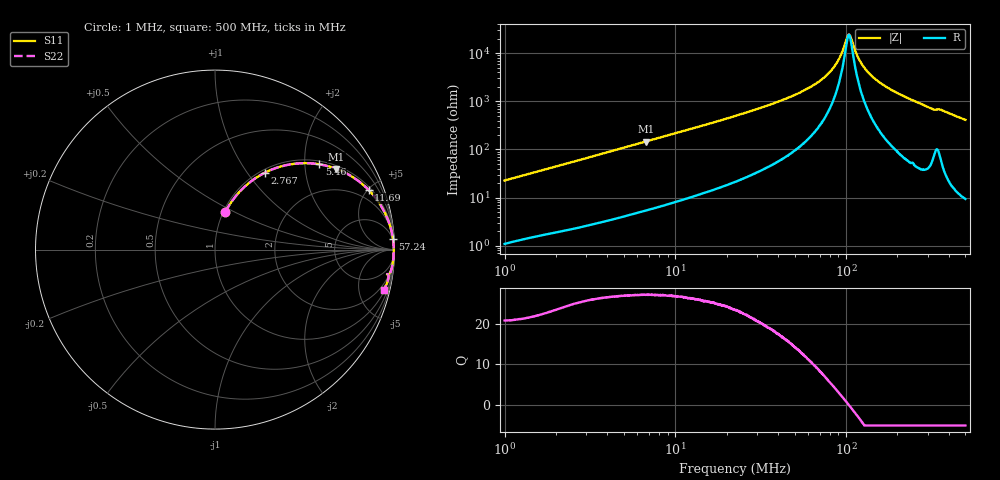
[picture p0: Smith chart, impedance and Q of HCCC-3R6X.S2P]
!s-Parameter Generated by FASTRON Sdn. Bhd.
!FASTRON P/N : HCCC-3R6X
!Keysight Technologies,E4991B,MY54100416,A.01.15
!Date: Thu Apr 02 14:45:55 2026
!Version  : Rev00 Thu Apr 02 14:45:55 2026
!Data & Calibration Information:
!PortZ  Port1:50+j0  Port2:50+j0
!When reading, reference impedance value at option line is always used.
!Remarks : This data is being provided solely for informational purposes.
!Freq	S11	S21	S12	S22
# Hz S dB R 50
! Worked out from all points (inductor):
!   1601 points, 1 MHz to 500 MHz, reference 50 ohm
!   read as one part in series: L = 3.57 uH near 1.032 MHz
!   highest Q = 27.1 at 6.76 MHz (marker M1), where L = 3.45 uH
!   self-resonance near 103.7 MHz
!   S11 on the Smith chart (normalised r, x): 1 MHz: 1.02, +0.45; 2.767 MHz: 1.05, +1.22; 5.46 MHz: 1.09, +2.37; 11.69 MHz: 1.19, +5.05; 57.24 MHz: 4, +34; 500 MHz: 1.19, -8.26
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1000000  -13.20 74.6  -0.31 -12.6  -0.31 -12.6  -13.20 74.6
2766663  -5.84 57.0  -1.52 -30.7  -1.52 -30.7  -5.84 57.0
2820919  -5.72 56.6  -1.56 -31.2  -1.56 -31.2  -5.72 56.6
5459542  -2.49 39.2  -3.97 -48.6  -3.97 -48.6  -2.49 39.2
6759791  -1.81 33.6  -5.12 -54.2  -5.12 -54.2  -1.81 33.6
7957584  -1.40 29.6  -6.12 -58.3  -6.12 -58.3  -1.40 29.6
1.168907e7  -0.74 21.3  -8.80 -66.5  -8.80 -66.5  -0.74 21.3
2.236068e7  -0.25 11.3  -14.14 -76.2  -14.14 -76.2  -0.25 11.3
5.72406e7  -0.06 3.3  -24.70 -81.9  -24.70 -81.9  -0.06 3.3
6.307767e7  -0.05 2.7  -26.34 -81.8  -26.34 -81.8  -0.05 2.7
7.483371e7  -0.04 1.8  -30.11 -80.2  -30.11 -80.2  -0.04 1.8
8.47377e7  -0.04 1.1  -34.18 -76.4  -34.18 -76.4  -0.04 1.1
9.158278e7  -0.04 0.7  -38.07 -69.7  -38.07 -69.7  -0.04 0.7
1.013146e8  -0.04 0.1  -46.46 -30.4  -46.46 -30.4  -0.04 0.1
1.04107e8  -0.04 -0.0  -47.83 2.2  -47.83 2.2  -0.04 -0.0
1.069764e8  -0.04 -0.2  -46.28 33.0  -46.28 33.0  -0.04 -0.2
1.178853e8  -0.04 -0.7  -38.12 70.7  -38.12 70.7  -0.04 -0.7
1.289013e8  -0.04 -1.2  -33.71 77.6  -33.71 77.6  -0.04 -1.2
1.476717e8  -0.04 -1.9  -29.39 81.5  -29.39 81.5  -0.04 -1.9
1.77937e8  -0.05 -3.1  -25.43 82.8  -25.43 82.8  -0.05 -3.1
3.149446e8  -0.17 -7.9  -17.20 78.0  -17.20 78.0  -0.17 -7.9
5e8  -0.29 -13.5  -12.61 75.2  -12.61 75.2  -0.29 -13.5
